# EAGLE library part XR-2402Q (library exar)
V.22bis high perfomance AFE
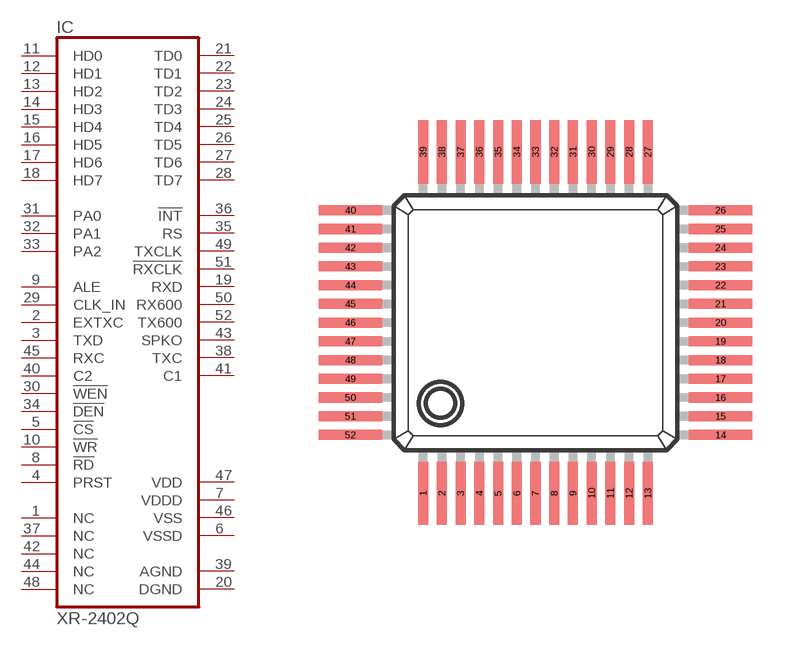
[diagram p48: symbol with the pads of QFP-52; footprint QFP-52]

Designator prefix IC

## XR-2402Q (OC_FARNELL: unknown; OC_NEWARK: unknown)  [QFP-52]
1  NC  nc
2  EXTXC  in
3  TXD  in
4  PRST  in
5  !CS  in
6  VSSD  pwr
7  VDDD  pwr
8  !RD  in
9  ALE  in
10  !WR  in
11  HD0
12  HD1
13  HD2
14  HD3
15  HD4
16  HD5
17  HD6
18  HD7
19  RXD  out
20  DGND  pwr
21  TD0
22  TD1
23  TD2
24  TD3
25  TD4
26  TD5
27  TD6
28  TD7
29  CLK_IN  in
30  !WEN  in
31  PA0  in
32  PA1  in
33  PA2  in
34  !DEN  in
35  RS  out
36  !INT  out
37  NC  nc
38  TXC  out
39  AGND  pwr
40  C2  in
41  C1  out
42  NC  nc
43  SPKO  out
44  NC  nc
45  RXC  in
46  VSS  pwr
47  VDD  pwr
48  NC  nc
49  TXCLK  out
50  RX600  out
51  !RXCLK  out
52  TX600  out

## Footprint QFP-52 (pad centres in mm)
Quad Flat Package
smd 0.35 x 2.2: 1 -3.575,-6.25; 2 -2.925,-6.25; 3 -2.275,-6.25; 4 -1.625,-6.25; 5 -0.975,-6.25; 6 -0.325,-6.25; 7 0.325,-6.25; 8 0.975,-6.25; 9 1.625,-6.25; 10 2.275,-6.25; 11 2.925,-6.25; 12 3.575,-6.25; 13 4.225,-6.25; 27 4.225,5.6; 28 3.575,5.6; 29 2.925,5.6; 30 2.275,5.6; 31 1.625,5.6; 32 0.975,5.6; 33 0.325,5.6; 34 -0.325,5.6; 35 -0.975,5.6; 36 -1.625,5.6; 37 -2.275,5.6; 38 -2.925,5.6; 39 -3.575,5.6
smd 2.2 x 0.35: 14 6.75,-4.225; 15 6.75,-3.575; 16 6.75,-2.925; 17 6.75,-2.275; 18 6.75,-1.625; 19 6.75,-0.975; 20 6.75,-0.325; 21 6.75,0.325; 22 6.75,0.975; 23 6.75,1.625; 24 6.75,2.275; 25 6.75,2.925; 26 6.75,3.575; 40 -6.1,3.575; 41 -6.1,2.925; 42 -6.1,2.275; 43 -6.1,1.625; 44 -6.1,0.975; 45 -6.1,0.325; 46 -6.1,-0.325; 47 -6.1,-0.975; 48 -6.1,-1.625; 49 -6.1,-2.275; 50 -6.1,-2.925; 51 -6.1,-3.575; 52 -6.1,-4.225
